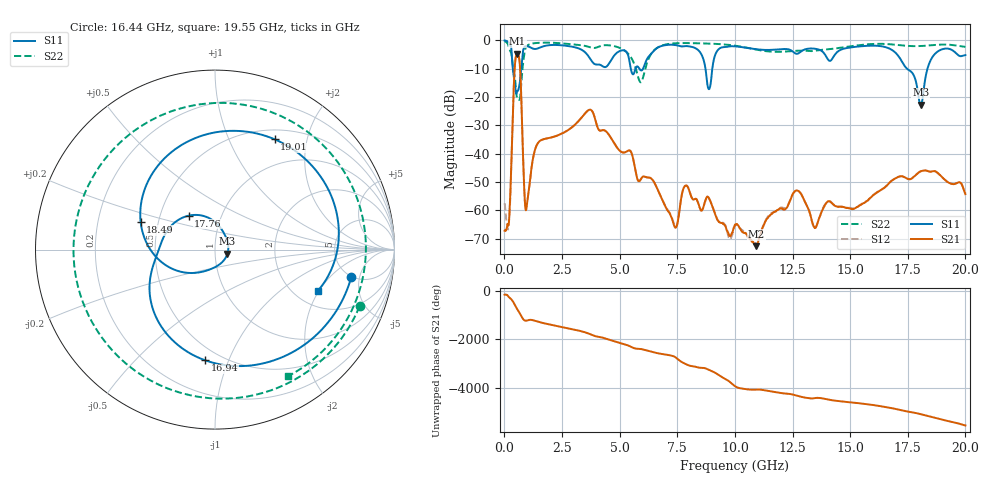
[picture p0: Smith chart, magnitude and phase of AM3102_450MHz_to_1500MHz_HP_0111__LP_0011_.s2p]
!Agilent Technologies,E8364B,MY43040894,A.07.50.67
!Agilent E8364B: A.07.50.67
!Date: Thursday, January 11, 2018 05:51:40
!Correction: S11(Full 2 Port(1,2))
!S21(Full 2 Port(1,2))
!S12(Full 2 Port(1,2))
!S22(Full 2 Port(1,2))
!S2P File: Measurements: S11, S21, S12, S22:
# Hz S  dB  R 50
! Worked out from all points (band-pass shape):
!   1601 points, 10 MHz to 20 GHz, reference 50 ohm
!   highest |S21| = -4.69 dB at 559.7 MHz (marker M1); lowest = -72.6 dB at 10.93 GHz (marker M2)
!   |S21| within 3 dB of the highest: 468.2 MHz to 661.7 MHz (193.6 MHz wide, 34.3 % of centre)
!   lowest |S11| = -22.7 dB at 18.06 GHz (marker M3), VSWR 1.16, Z = 57.4 - j2.58 ohm
!   |S11| at or under -10 dB: 366.2 MHz to 732 MHz (365.8 MHz wide, 66.6 % of centre); 8.724 GHz to 9.02 GHz (296 MHz wide, 3.34 % of centre); 17.46 GHz to 18.36 GHz (891.7 MHz wide, 4.98 % of centre)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
!   |S22| runs from -21.0 to -0.4 dB; largest |S21 - S12| = 0.0018
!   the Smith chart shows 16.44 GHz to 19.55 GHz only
!   S11 on the Smith chart (normalised r, x): 16.44 GHz: 4.90, -3.77; 16.94 GHz: 0.41, -0.83; 17.76 GHz: 0.70, +0.28; 18.49 GHz: 0.40, +0.15; 19.01 GHz: 0.62, +1.49; 19.55 GHz: 2.62, -1.95
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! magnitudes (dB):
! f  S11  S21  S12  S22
! 10 MHz  -0.1  -67.2  -57.4  -0.4
! 197.4 MHz  -0.7  -64.0  -64.4  -2.5
! 559.7 MHz  -18.0  -4.7  -4.7  -20.6
! 959.5 MHz  -2.0  -59.0  -58.9  -2.2
! 1.459 GHz  -2.8  -36.2  -36.2  -0.9
! 3.346 GHz  -3.3  -27.3  -27.3  -1.7
! 5.907 GHz  -10.5  -49.2  -49.1  -14.8
! 6.682 GHz  -2.4  -53.2  -53.2  -2.4
! 8.881 GHz  -17.2  -55.8  -55.7  -1.2
! 10.01 GHz  -2.1  -65.0  -65.3  -1.9
! 10.93 GHz  -3.2  -72.6  -71.7  -3.3
! 12.64 GHz  -4.7  -53.0  -53.1  -3.7
! 13.34 GHz  -2.9  -63.7  -63.8  -3.8
! 16.44 GHz  -2.2  -52.2  -52.2  -1.3
! 16.68 GHz  -2.8  -50.5  -50.4  -1.4
! 16.94 GHz  -4.2  -48.8  -48.8  -1.5
! 17.76 GHz  -12.4  -48.1  -48.2  -2.1
! 18.06 GHz  -22.7  -46.2  -46.2  -2.0
! 18.49 GHz  -7.1  -46.3  -46.3  -1.8
! 19.01 GHz  -3.1  -48.4  -48.5  -1.5
! 19.55 GHz  -4.2  -50.6  -50.5  -1.8
! 20 GHz  -5.2  -54.2  -53.9  -2.3
